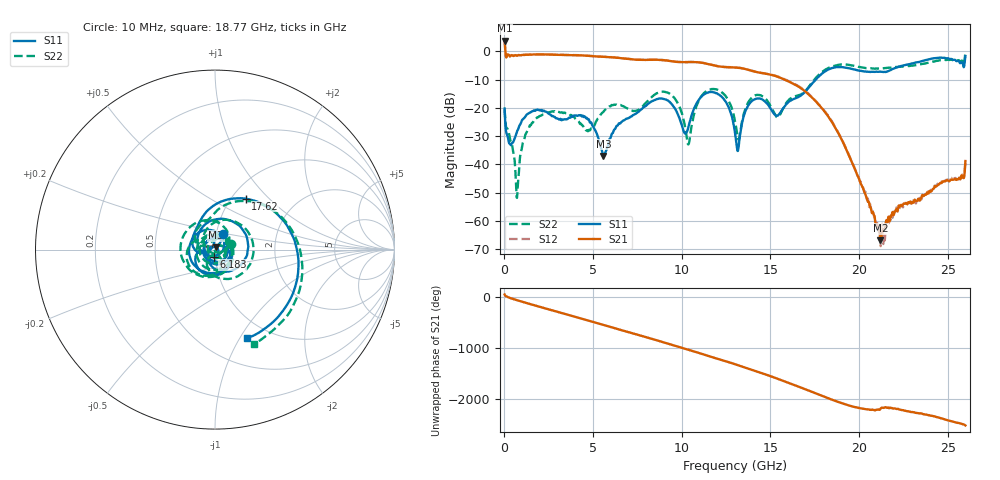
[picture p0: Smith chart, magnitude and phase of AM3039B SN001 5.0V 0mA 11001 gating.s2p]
!Agilent Technologies,E8364B,MY43040894,A.07.50.67
!Agilent E8364B: A.07.50.67
!Date: Tuesday, June 28, 2016 08:12:00
!Correction: S11(Full 2 Port(1,2))
!S21(Full 2 Port(1,2))
!S12(Full 2 Port(1,2))
!S22(Full 2 Port(1,2))
!S2P File: Measurements: S11, S21, S12, S22:
# Hz S  dB  R 50
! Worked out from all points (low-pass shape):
!   1601 points, 10 MHz to 26 GHz, reference 50 ohm
!   highest |S21| = 3.77 dB at 10 MHz (marker M1); lowest = -66.9 dB at 21.21 GHz (marker M2)
!   |S21| within 3 dB of the highest: start of sweep to 43.98 MHz
!   lowest |S11| = -37.1 dB at 5.582 GHz (marker M3), VSWR 1.03, Z = 50.5 + j1.31 ohm
!   |S11| at or under -10 dB: start of sweep to 17.56 GHz
!   |S22| runs from -51.9 to -0.3 dB; largest |S21 - S12| = 0.023
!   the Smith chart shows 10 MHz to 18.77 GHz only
!   S11 on the Smith chart (normalised r, x): 10 MHz: 1.08, +0.19; 6.183 GHz: 0.98, -0.08; 17.62 GHz: 1.16, +0.74; 18.77 GHz: 0.79, -1.08
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1e7  -20.25 62.1  3.77 41.0  3.83 41.8  -20.54 19.4
7.572125e8  -27.81 96.9  -1.43 -74.8  -1.39 -74.6  -47.17 132.3
1.731838e9  -21.07 4.6  -1.15 -173.5  -1.11 -173.3  -24.11 -21.1
2.803925e9  -23.16 -146.4  -1.22 80.9  -1.15 80.9  -21.30 -175.0
4.347081e9  -22.94 -51.2  -1.46 -71.0  -1.43 -70.8  -25.93 -64.7
5.581606e9  -37.06 67.1  -1.97 166.2  -1.91 166.3  -21.42 14.4
6.182625e9  -27.82 -101.2  -2.19 105.6  -2.14 105.7  -18.87 -80.8
7.303444e9  -22.50 68.9  -2.95 -6.0  -2.90 -5.9  -21.08 85.5
8.684162e9  -16.80 -142.9  -3.01 -144.8  -2.95 -144.6  -14.68 -155.0
9.772494e9  -22.19 57.1  -3.79 102.8  -3.74 102.9  -18.39 54.8
1.071463e10  -20.00 162.7  -3.82 4.7  -3.76 4.7  -21.81 141.8
1.160804e10  -14.43 36.8  -4.71 -93.8  -4.66 -93.9  -13.50 19.7
1.3005e10  -28.83 -159.4  -5.73 116.9  -5.69 116.7  -24.91 -127.2
1.734208e10  -11.53 84.5  -16.31 -65.3  -16.13 -65.0  -11.11 70.6
1.761822e10  -9.60 58.9  -18.11 -103.0  -17.93 -102.5  -9.02 47.2
1.877153e10  -5.59 -69.9  -28.32 104.2  -28.13 104.3  -4.88 -67.7
1.982738e10  -6.58 -178.4  -42.66 -7.6  -42.47 -8.7  -5.32 -169.3
2.120809e10  -7.24 71.6  -66.86 -38.9  -67.10 -58.1  -6.06 83.1
2.167916e10  -6.92 41.1  -58.76 -23.5  -60.82 -18.0  -5.86 47.8
2.3401e10  -3.74 -91.2  -52.85 -127.3  -52.13 -126.1  -4.67 -80.2
2.452182e10  -2.28 176.1  -47.01 148.1  -46.73 148.9  -3.24 -166.5
2.6e10  -1.74 3.8  -38.84 -3.1  -38.66 -6.1  -0.33 37.5
